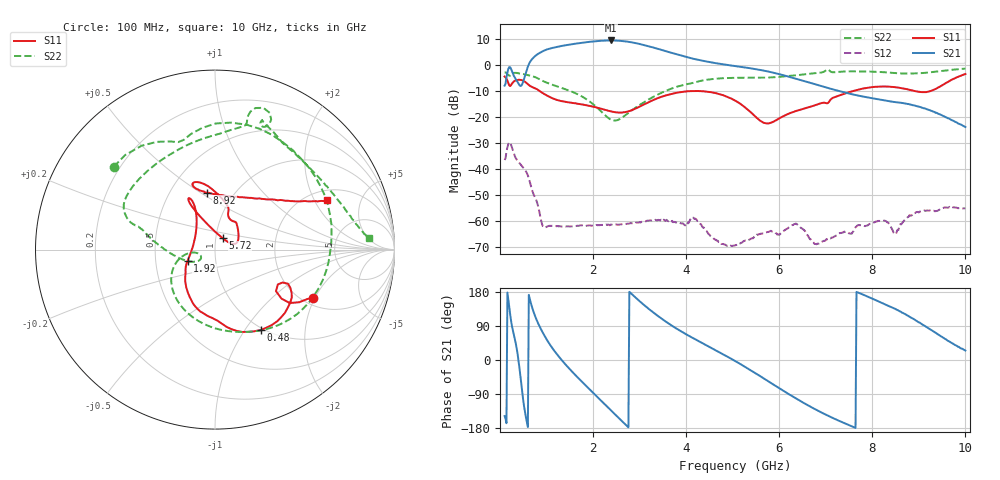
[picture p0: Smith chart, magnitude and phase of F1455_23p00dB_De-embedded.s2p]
! Integrated Device Technology
! Corporate Headquarters
! 6024 Silver Creek Valley Road
! San Jose, CA 95138  USA
! Phone:  1-408-284-8200
! Toll Free:  1-800-223-1366
! Webpage:  http://www.idt.com/
! Timing and RF Division
! 515 Groton Road, Suite 102
! Westford, MA 01886-6024
! Device:  F1455
! Description: 6-bit 0.5 dB Transmit Variable Gain Amplifier
! Frequency:  1400.0 -  2300.00 MHz
! Package:  6x6 mm Thin QFN Plastic Package: 28 pin
! State:  46
! Atten State:  23.0 dB
! Voltage:  +5.00 Volts
! Current:  217.644 mA
! Data:  The device was measured on a the F1455 evaluation board which has
!  individual transmission lines to the RF pins.  Data was collected
!  using a calibrated network analyzer.  The evaluation board was
!  de-embedded using a TRL calibration technique.
!  The reference plane is the edge of the package pin.
!  Pin  1 = CSb
!  Pin  2 = DATA
!  Pin  3 = CLK
!  Pin  4 = RSET
!  Pin  5 = GND
!  Pin  6 = RFIN  = Port 1
!  Pin  7 = GND
!  Pin  8 = NC
!  Pin  9 = NC
!  Pin 10 = NC
!  Pin 11 = NC
!  Pin 12 = NC
!  Pin 13 = NC
!  Pin 14 = /STBY
!  Pin 15 = GND
!  Pin 16 = RFOUT  = Port 2
!  Pin 17 = GND
!  Pin 18 = NC
!  Pin 19 = NC
!  Pin 20 = NC
!  Pin 21 = GND
!  Pin 22 = NC
!  Pin 23 = GND
!  Pin 24 = NC
!  Pin 25 = NC
!  Pin 26 = NC
!  Pin 27 = GND
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# GHz S dB R 50
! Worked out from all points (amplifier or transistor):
!   496 points, 100 MHz to 10 GHz, reference 50 ohm
!   highest |S21| = 9.6 dB at 2.38 GHz (marker M1)
!   |S21| within 3 dB of that: 1.099 GHz to 3.35 GHz (2.252 GHz wide, 101 % of centre)
!   unconditionally stable (mu >= 1): start of sweep to end of sweep
!   at 1.74 GHz: K = 198.82, MAG = 9.1 dB, |S12| = -61.5 dB
!   at 5.06 GHz: K = 945.76, MAG = 1.7 dB, |S12| = -69.1 dB
!   at 10 GHz: K = 589.79, MAG = -15.1 dB, |S12| = -55.0 dB
!   S11 on the Smith chart (normalised r, x): 100 MHz: 2.27, -1.93; 480 MHz: 0.97, -1.18; 1.92 GHz: 0.73, -0.10; 5.72 GHz: 1.08, +0.14; 8.92 GHz: 0.76, +0.53; 10 GHz: 2.45, +2.52
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0.1  -4.31 -26.1  -7.80 -147.9  -36.37 47.2  -2.75 140.7
0.18  -6.74 -36.4  -1.35 160.1  -30.22 -6.8  -3.70 112.6
0.26  -6.95 -25.1  -2.36 88.0  -31.74 -77.0  -3.32 95.9
0.38  -5.59 -42.2  -6.47 15.1  -36.72 -118.1  -3.00 58.0
0.48  -5.76 -60.4  -7.19 -86.9  -38.90 -149.6  -3.28 31.5
0.68  -8.22 -90.4  2.18 143.1  -47.31 138.0  -4.09 -15.5
0.82  -9.46 -108.8  4.42 96.7  -54.18 109.0  -5.05 -46.5
0.96  -11.12 -123.6  5.75 63.4  -62.41 127.2  -6.32 -71.9
1.34  -13.79 -143.6  7.51 -2.1  -61.94 104.4  -8.76 -121.7
1.76  -14.99 -153.4  8.67 -57.2  -61.50 72.8  -11.95 -156.5
1.92  -15.59 -156.9  9.02 -76.6  -61.53 64.7  -13.80 -165.6
2.38  -17.65 -177.4  9.56 -132.3  -61.22 49.0  -20.84 -163.4
2.8  -17.43 144.8  8.94 177.6  -60.66 40.1  -17.74 -148.6
3.1  -14.99 125.1  7.78 144.6  -59.96 32.1  -14.15 -165.3
3.4  -12.56 116.9  6.31 115.6  -59.37 20.0  -11.18 -179.7
4.08  -9.92 116.3  2.83 62.4  -59.53 6.9  -7.01 163.2
5.06  -13.62 114.8  -0.29 -3.2  -69.14 11.9  -4.79 147.9
5.72  -22.29 55.9  -2.22 -52.7  -64.24 17.3  -4.71 120.9
6.7  -15.78 37.2  -6.89 -125.2  -67.41 -133.4  -3.15 78.4
8.36  -8.19 108.4  -13.78 142.0  -60.94 76.5  -2.79 62.3
8.92  -9.90 97.8  -15.48 105.6  -56.78 102.5  -3.13 39.8
10  -3.35 23.9  -23.71 24.9  -55.00 29.9  -1.28 4.5
